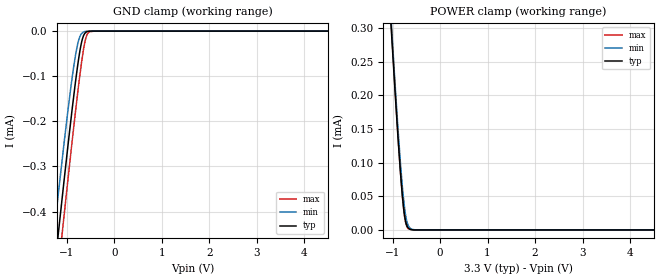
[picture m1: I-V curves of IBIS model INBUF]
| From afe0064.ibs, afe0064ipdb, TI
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|   INBUF Model
[Model] INBUF
|Signals SMT-MD(98), STI(97), PGA-x(94-96), INTUPZ(93), ENTRI(92), NAPZ(89),
|   PDZ(88), DF-SM(72), CLK(70), SHR(69), SHS(68), IRST(67), INTG(66)
Model_type Input
Vinl = 0.66
Vinh = 2.64
|   typ   min   max
|   (nom PVT)   (Fast PVT)   (slow PVT)
C_comp   3.1005860e-13   3.1004500e-13   3.1397710e-13
| Where   nom PVT is  Weak Process, 3.3V, 37C
|   Fast PVT is Nominal Process, 3.4V, 0C
|   Slow PVT is Strong Process, 3.2V, 95C
| variable   typ   min   max
[Voltage Range]   3.3   3.2   3.4
[Temperature Range]   37   95   0
|Operating temp range   27   85   0
[Power Clamp Reference]   3.3   3.2   3.4
[GND Clamp Reference]   0   0   0
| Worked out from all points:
|   GND clamp passes 1 mA (typ) near -1.73 V on its own axis
|   POWER clamp passes 1 mA (typ) near -1.58 V on its own axis
[GND Clamp]
|   Voltage   I(typ)   I(min)   I(max)
-3.3V     -2.613mA   -2.494mA   -2.717mA
-1.266V   -536.8uA   -446uA     -619.1uA
-1.181V   -453.3uA   -365.5uA   -534.4uA
-1.162V   -434.8uA   -347.7uA   -515.5uA
-1.09V    -364.9uA   -280.5uA   -443.3uA
-914.3mV  -199.4uA   -126.1uA   -271.8uA
-808.6mV  -107.4uA   -49.76uA   -172.6uA
-724.9mV  -45.78uA   -12.89uA   -99.54uA
-644.9mV  -10.06uA   -1.912uA   -39.8uA
-564mV    -1.042uA   -328.5nA   -6.395uA
-414.5mV  -45.33nA   -61.82nA   -22.22nA
6.6V      0A         0A         0A
[POWER Clamp]
|   Voltage   I(typ)   I(min)   I(max)
-3.3V     3.258mA    3.253mA    3.275mA
-1.025V   297.5uA    307.2uA    303.9uA
-1.017V   287.6uA    297.7uA    293.8uA
-1.013V   283.2uA    293.4uA    289.3uA
-883.3mV  136.2uA    148.8uA    139.2uA
-825.4mV  79.27uA    92.64uA    79.58uA
-797mV    54.43uA    68.07uA    54.54uA
-743.3mV  20.39uA    31.18uA    18.43uA
-707.1mV  8.433uA    15.41uA    6.782uA
-665.6mV  2.706uA    6.104uA    1.743uA
-503.3mV  48.65nA    67.72nA    31.18nA
6.6V      0A         0A         0A
